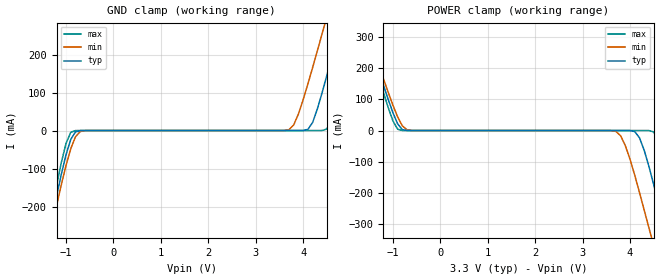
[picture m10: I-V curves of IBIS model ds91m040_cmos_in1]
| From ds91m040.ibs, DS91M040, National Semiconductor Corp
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|   Model  ds91m040_cmos_in1
[Model]   ds91m040_cmos_in1
Model_type Input
Vinh=2.0
Vinl=0.8
|   Typ   Min   Max
C_comp   1.823pF   1.78pf   1.867pF
[Model Spec]
S_overshoot_high   3.3   3.0   3.6
S_overshoot_low   0.0   0.0   0.0
[Temperature Range]   25   85   -40
[Voltage Range]   3.3   3.0   3.6
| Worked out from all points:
|   GND clamp passes 1 mA (typ) near -0.72 V on its own axis
|   POWER clamp passes 1 mA (typ) near -0.73 V on its own axis
[GND Clamp]
-3.3V     -1.413A    -1.366A    -1.475A
-1.4V     -294.4mA   -311.8mA   -275.9mA
-1.3V     -233.9mA   -255.1mA   -210.4mA
-1V       -63.76mA   -91.86mA   -33.88mA
-800mV    -3.538mA   -16.33mA   -127.5uA
3.7V      2.508uA    2.179mA    5.038uA
4.1V      2.974mA    122.6mA    5.039uA
4.4V      99.8mA     255.1mA    78.96uA
4.5V      145.1mA    300.5mA    4.129mA
4.8V      287.3mA    438.7mA    121.9mA
5.1V      433.3mA    578.6mA    273.4mA
6.5V      1.128A     1.24A      1.009A
[POWER Clamp]
-3.3V     1.178A     1.145A     1.062A
-1.6V     335.7mA    346.3mA    325mA
-900mV    21.35mA    43.51mA    4.129mA
-600mV    5.631uA    137.7uA    5.046uA
3.7V      -1.11uA    -2.689mA   -420.4nA
3.9V      -10.67uA   -47.87mA   -1.298uA
4.2V      -23.42mA   -198.5mA   -2.695uA
4.4V      -115.6mA   -311.8mA   -127.5uA
4.5V      -173.5mA   -368.3mA   -4.73mA
4.8V      -354.8mA   -537.4mA   -145.6mA
5.1V      -535mA     -705.2mA   -341.2mA
6.5V      -1.355A    -1.366A    -1.229A
